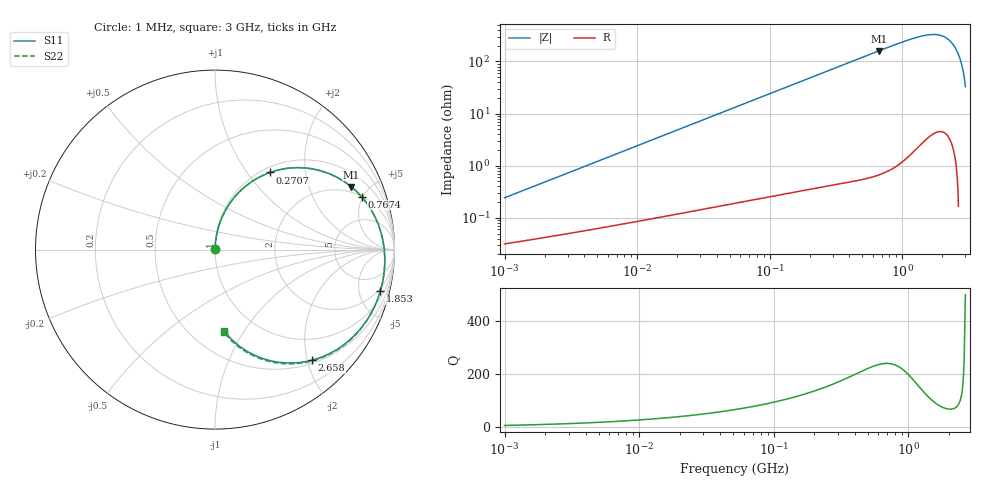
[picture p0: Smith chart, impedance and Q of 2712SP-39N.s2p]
# MHz  S  MA  R  50
!Freq  MagS11  AngS11  MagS21  AngS21  MagS12  AngS12  MagS22  AngS22
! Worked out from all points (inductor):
!   801 points, 1 MHz to 3 GHz, reference 50 ohm
!   read as one part in series: L = 38.4 nH near 1.041 MHz
!   highest Q = 241 at 667 MHz (marker M1), where L = 38.2 nH
!   S11 on the Smith chart (normalised r, x): 1 MHz: 1.00, +0.00; 270.7 MHz: 1.08, +1.29; 767.4 MHz: 2.04, +4.90; 1.853 GHz: 1.62, -7.73; 2.658 GHz: 0.56, -2.09; 3 GHz: 0.72, -0.82
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1  0.002327 82.1  0.9997 -0.1  0.9997 -0.1  0.002327 82.1
3.829105  0.008842 85.9  0.9994 -0.6  0.9994 -0.6  0.008841 85.9
14.51587  0.03344 86.2  0.9984 -2.1  0.9984 -2.1  0.03343 86.2
55.02866  0.1257 81.3  0.9902 -7.9  0.9902 -7.9  0.1256 81.3
117.8422  0.2616 72.8  0.9625 -16.6  0.9625 -16.6  0.2615 72.8
208.6098  0.4324 61.4  0.8985 -28.1  0.8985 -28.1  0.4322 61.4
270.6905  0.5283 54.5  0.8458 -35.1  0.8458 -35.1  0.5279 54.5
429.1813  0.7021 39.9  0.7088 -49.8  0.7088 -49.8  0.7015 39.9
666.9689  0.8368 24.7  0.5445 -65.1  0.5445 -65.1  0.8359 24.7
767.4077  0.8686 19.8  0.4923 -69.9  0.4923 -69.9  0.8677 19.8
790.8254  0.8747 18.8  0.4815 -71.0  0.4815 -71.0  0.8737 18.8
1253.858  0.9382 2.6  0.3395 -87.0  0.3395 -87.0  0.9372 2.6
1563.078  0.9502 -6.1  0.2996 -95.4  0.2996 -95.4  0.9495 -6.1
1853.343  0.95 -14.1  0.2939 -103.3  0.2939 -103.3  0.9496 -14.1
2090.131  0.9406 -21.4  0.3155 -110.5  0.3155 -110.5  0.941 -21.5
2310.405  0.9195 -29.6  0.3653 -118.7  0.3653 -118.7  0.9209 -29.6
2503.225  0.8805 -38.8  0.4438 -128.1  0.4438 -128.1  0.8833 -38.9
2658.329  0.8201 -48.7  0.541 -138.1  0.541 -138.1  0.8244 -48.7
2823.044  0.6986 -62.8  0.6838 -152.5  0.6838 -152.5  0.7053 -62.9
2909.189  0.5971 -72.3  0.7706 -162.1  0.7706 -162.1  0.6052 -72.3
2997.964  0.4579 -83.5  0.858 -173.5  0.858 -173.5  0.4674 -83.6
3000  0.4543 -83.8  0.8599 -173.7  0.8599 -173.7  0.4638 -83.9
